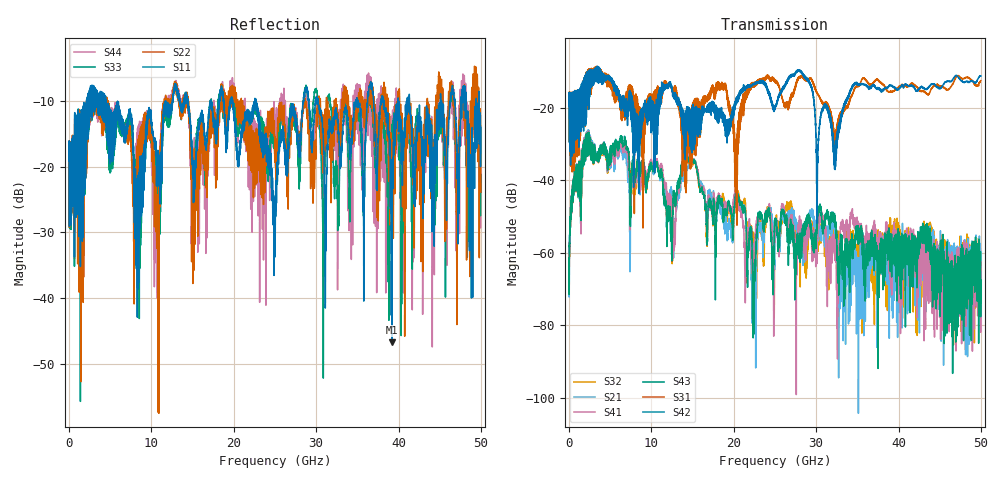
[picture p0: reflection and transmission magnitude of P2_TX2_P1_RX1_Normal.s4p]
!Keysight Technologies,N5225B,MY57041031,A.13.20.10
!Date: Friday, May 31, 2019 11:14:35
!Correction: S11(Full 4 Port(1,2,3,4))
!S12(Full 4 Port(1,2,3,4))
!S13(Full 4 Port(1,2,3,4))
!S14(Full 4 Port(1,2,3,4))
!S21(Full 4 Port(1,2,3,4))
!S22(Full 4 Port(1,2,3,4))
!S23(Full 4 Port(1,2,3,4))
!S24(Full 4 Port(1,2,3,4))
!S31(Full 4 Port(1,2,3,4))
!S32(Full 4 Port(1,2,3,4))
!S33(Full 4 Port(1,2,3,4))
!S34(Full 4 Port(1,2,3,4))
!S41(Full 4 Port(1,2,3,4))
!S42(Full 4 Port(1,2,3,4))
!S43(Full 4 Port(1,2,3,4))
!S44(Full 4 Port(1,2,3,4))
!S4P File: Measurements: <S11,S12,S13,S14>,
!<S21,S22,S23,S24>,
!<S31,S32,S33,S34>,
!<S41,S42,S43,S44>:
# Hz S  dB  R 50.0
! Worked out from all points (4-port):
!   5000 points, 10 MHz to 50 GHz, reference 50 ohm
!   strongest paths, dB at 10 MHz, 12.51 GHz, 25.01 GHz, 37.51 GHz, 50 GHz:
!     S42: -19.5, -14.8, -19.9, -14.6, -11.3
!     S31: -19.4, -14.9, -13.0, -12.4, -12.6
!     S43: -61.5, -58.2, -50.6, -68.4, -73.9
!     S41: -70.2, -47.8, -54.1, -56.1, -63.2
!     S21: -63.5, -45.2, -56.0, -60.5, -68.0
!     S32: -61.3, -57.1, -52.7, -56.8, -73.5
!   lowest |S11| = -46.8 dB at 39.22 GHz (marker M1), VSWR 1.01, Z = 50 + j0.456 ohm
!   |S11| at or under -10 dB: 4.481 GHz to 11.72 GHz (7.238 GHz wide, 89.4 % of centre); 22.72 GHz to 28.43 GHz (5.704 GHz wide, 22.3 % of centre); 30.26 GHz to 34.82 GHz (4.559 GHz wide, 14 % of centre)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
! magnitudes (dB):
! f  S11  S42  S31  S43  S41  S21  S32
! 10 MHz  -19.1  -19.5  -19.4  -61.5  -70.2  -63.5  -61.3
! 2.26 GHz  -13.5  -15.7  -12.5  -27.3  -27.0  -26.7  -27.1
! 20.24 GHz  -14.5  -17.5  -32.3  -44.1  -43.4  -44.5  -43.9
! 22.46 GHz  -10.7  -13.6  -13.8  -69.2  -59.3  -58.4  -55.1
! 32.27 GHz  -12.1  -31.5  -30.4  -49.9  -58.4  -52.3  -55.8
! 39.22 GHz  -46.8  -13.9  -15.7  -62.2  -62.5  -59.0  -53.0
! 50 GHz  -14.0  -11.3  -12.6  -73.9  -63.2  -68.0  -73.5
